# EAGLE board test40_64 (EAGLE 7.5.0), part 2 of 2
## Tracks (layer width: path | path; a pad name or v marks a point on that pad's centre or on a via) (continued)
L2 (continued)
  Top 0.51: J18.2 194.4,280.52 195.75,281.88 324.5,281.88 328,278.38 330,278.38 331.12,279.5 331.49,279.5 J9.2
L3
  Top 0.406: X1.12 26.01,253.89 56.25,284.12 108.12,284.12 114.62,277.62 115.73,277.62 J7.3 116.57,277.57 117.88,278.88 126,278.88 127.12,277.75 127.7,277.75 J17.3 128.44,277.69 129.75,279 178,279 179.25,277.75 180.21,277.75 J8.3 181.05,277.68 182.38,279 189.75,279 191,277.75 191.78,277.75 J18.3
  Top 0.506: J9.3 329.88,277.12 331.12,278.38 340,278.38 341.25,277.12 J19.3 342.88,277.12 344.12,278.38 345.5,278.38 348,280.88 475.38,280.88 478.62,277.62 479.86,277.62 J10.3 480.58,277.7 482,279 490,279 491.38,277.62 492.06,277.62 J20.3
  Top 0.51: J18.3 192.55,277.68 193.88,279 195.12,279 197.12,281 242.88,281 245,278.88 325.88,278.88 327.62,277.12 J9.3
L4
  Top 0.406: X1.31 26.37,252.49 30.12,256.25 30.25,256.25 57,283 107.88,283 114.5,276.38 116.5,276.38 117.75,277.62 118.27,277.62 J7.4 126.06,277.57 127.25,276.38 128.25,276.38 129.5,277.62 130.22,277.62 J17.4 177.93,277.69 179.25,276.38 180.88,276.38 182.12,277.62 182.78,277.62 J8.4 189.7,277.68 191,276.38 192.38,276.38 193.62,277.62 194.35,277.62 J18.4
  Top 0.506: J9.4 340,277.12 341.25,275.88 343.12,275.88 344.25,277 344.73,277 J19.4 346.38,277.12 347.75,278.5 408.25,278.5 408.38,278.38 476.25,278.38 478.25,276.38 480.62,276.38 481.88,277.62 482.39,277.62 J10.4 482.52,277.75 489.88,277.75 491.25,276.38 493.12,276.38 494.45,277.7 J20.4
  Top 0.51: J9.4 331.12,277.12 329.88,275.88 326.25,275.88 325.88,276.25 245.38,276.25 243.88,277.75 194.47,277.75 J18.4
L5
  Top 0.406: X1.13 26.5,251.12 57.5,282.12 107.25,282.12 114.25,275.12 115.69,275.12 J7.5 116.41,275.03 117.62,276.25 126.12,276.25 127.25,275.12 127.72,275.12 J17.5 128.53,275.15 129.88,276.5 178,276.5 179.38,275.12 J8.5 180.88,275.13 182.12,276.38 189.62,276.38 190.88,275.12 J18.5
  Top 0.506: J9.5 329.83,274.58 331.12,275.88 340.12,275.88 341.5,274.5 342.23,274.5 J19.5 342.35,274.62 343.12,274.62 344.38,275.88 477,275.88 477.71,275.17 J10.5 480.67,275.17 481.88,276.38 489.75,276.38 490.88,275.25 492.05,275.25 J20.5
  Top 0.51: J18.5 192.26,275.13 193.5,276.38 242.5,276.38 245.12,273.75 262,273.75 263.12,274.88 325.88,274.88 326.25,274.5 329.02,274.5 J9.5
L6
  Top 0.406: X1.32 26.72,249.72 56.5,279.5 79.25,279.5 79.38,279.38 108.75,279.38 114.5,273.62 116.25,273.62 117.62,275 118.3,275 J7.6 126.09,275.03 127.25,273.88 128.5,273.88 129.62,275 130.14,275 J17.6 178.09,275.15 179.38,273.88 181,273.88 182.25,275.12 182.81,275.12 J8.6 189.49,275.13 190.75,273.88 192.25,273.88 193.38,275 194.26,275 J18.6
  Top 0.506: J9.6 340.17,274.58 341.5,273.25 343,273.25 344.25,274.5 344.76,274.5 J19.6 407.42,274.58 408.75,273.25 427.88,273.25 428.5,273.88 480.75,273.88 482,275.12 482.44,275.12 J10.6 489.58,275.17 490.88,273.88 492.88,273.88 494.12,275.12 494.63,275.12 J20.6
  Top 0.51: J9.6 331.21,274.58 330,273.38 264.38,273.38 262.25,271.25 245.5,271.25 241.62,275.12 J18.6
L7
  Top 0.406: X1.14 27.35,248.35 55.88,277.12 109.62,276.88 114,272.5 115.78,272.5 J7.7 116.36,272.49 117.62,273.75 126,273.75 127.12,272.62 127.75,272.62 J17.7 128.49,272.62 129.75,273.88 178.12,273.88 179.5,272.5 180.19,272.5 J8.7 181.09,272.6 182.38,273.88 189.62,273.88 190.88,272.62 191.83,272.62 J18.7
  Top 0.506: J9.7 329.8,272.05 331,273.25 340.25,273.25 341.5,272 342.26,272 J19.7 343.05,272.05 344.25,273.25 406.38,273.25 408.88,270.75 427,270.75 428.62,272.38 479.69,272.38 J10.7 480.62,272.62 481.88,273.88 489.62,273.88 490.88,272.62 J20.7
  Top 0.51: J18.7 192.34,272.6 193.62,273.88 240,273.88 245.25,268.62 262.38,268.62 265.88,272.12 329.03,272.12 J9.7
L8
  Top 0.406: X1.33 27.23,246.98 54.75,274.5 110,274.5 113.38,271.12 116.5,271.12 117.75,272.38 118.21,272.38 J7.8 126.01,272.49 127.12,271.38 128.38,271.38 129.62,272.62 130.28,272.62 J17.8 178.13,272.62 179.5,271.25 180.75,271.25 182,272.5 182.73,272.5 J8.8 189.53,272.6 190.88,271.25 192.38,271.25 193.62,272.5 194.31,272.5 J18.8
  Top 0.506: J9.8 340.2,272.05 341.5,270.75 342.88,270.75 344.12,272 344.81,272 J19.8 345.06,272.25 404.25,272.25 408.25,268.25 425.88,268.25 429,271.38 480.75,271.38 482,272.62 J10.8 489.5,272.62 490.88,271.38 492.75,271.38 494.12,272.62 J20.8
  Top 0.51: J9.8 331.17,272.05 329.88,270.75 267.25,270.75 262.62,266.12 245.38,266.12 238.88,272.62 194.43,272.62 J18.8
L9
  Top 0.406: X1.15 27.33,245.58 53.5,271.88 111.38,271.88 113.25,270 115.73,270 J7.9 116.58,269.95 117.88,271.25 126,271.25 127.12,270.12 127.7,270.12 J17.9 128.32,270.07 129.62,271.38 178.12,271.38 179.38,270.12 180.22,270.12 J8.9 180.68,270.06 182,271.38 189.75,271.38 191.12,270 191.81,270 J18.9 | 482,271.38 489.38,271.38 489.5,271.25
  Top 0.506: J9.9 329.88,269.5 331.12,270.75 340.12,270.75 341.38,269.5 J19.9 342.88,269.5 344.12,270.75 403.75,270.75 408.88,265.62 425,265.62 429.38,270 479.85,270 J10.9 480.71,270.08 482,271.38 | 489.5,271.25 490.62,270.12 492.1,270.12 J20.9
  Top 0.51: J18.9 192.43,270.06 193.75,271.38 237.25,271.38 245,263.62 261.88,263.62 267.75,269.5 J9.9
L10
  Top 0.406: X1.34 27.34,244.21 52.75,269.5 112,269.25 112.62,268.62 116.38,268.62 117.62,269.88 118.25,269.88 J7.10 126.05,269.95 127.12,268.88 128.25,268.88 129.5,270.12 130.25,270.12 J17.10 178.18,270.07 179.5,268.75 180.75,268.75 182,270 182.77,270 J8.10 189.82,270.06 191.12,268.75 192.25,268.75 193.5,270 194.34,270 J18.10
  Top 0.506: J9.10 340,269.5 341.25,268.25 342.88,268.25 344.12,269.5 J19.10 402.62,269.5 409,263.12 425.25,263.12 430.88,268.75 480.62,268.75 481.96,270.08 J10.10 489.29,270.08 490.5,268.88 493.46,268.88 J20.10
  Top 0.51: J9.10 331.13,269.5 329.88,268.25 268.38,268.25 261.12,261 245.62,261 236.38,270.25 194.59,270.25 J18.10
L11
  Top 0.406: X1.16 27.71,242.84 51.75,266.88 86.25,266.88 86.88,267.5 115.69,267.5 J7.11 116.53,267.41 117.75,268.62 126.12,268.62 127.25,267.5 127.72,267.5 J17.11 128.28,267.54 129.5,268.75 178.25,268.75 179.38,267.62 180.18,267.62 J8.11 181.01,267.51 182.25,268.75 189.88,268.75 191.12,267.5 191.84,267.5 J18.11
  Top 0.506: J9.11 329.84,266.96 331.12,268.25 340,268.25 341.25,267 342.27,267 J19.11 342.84,266.96 344.12,268.25 401.12,268.25 408.88,260.62 425.25,260.62 432.12,267.5 479.89,267.5 J10.11 480.67,267.55 482,268.88 489.25,268.88 490.75,267.38 491.96,267.38 J20.11
  Top 0.51: J18.11 192.39,267.51 193.62,268.75 235,268.75 245.25,258.5 261.12,258.5 269.62,267 329.07,267 J9.11
L12
  Top 0.406: X1.35 28.19,241.44 51,264.25 85.75,264.25 87.62,266.12 116.38,266.12 117.62,267.38 118.29,267.38 J7.12 126.09,267.41 127.25,266.25 128.5,266.25 129.75,267.5 130.26,267.5 J17.12 178.22,267.54 179.5,266.25 180.88,266.25 182.12,267.5 182.81,267.5 J8.12 189.74,267.51 191,266.25 192.38,266.25 193.5,267.38 194.26,267.38 J18.12
  Top 0.506: J9.12 339.91,266.96 341.12,265.75 343,265.75 344.25,267 344.81,267 J19.12 399.91,266.96 408.75,258.12 421.12,258.12 421.25,258 424.75,258 432.88,266.38 479,266.38 479.12,266.25 480.62,266.25 481.75,267.38 482.31,267.38 J10.12 489.2,267.55 490.5,266.25 492.62,266.25 493.75,267.38 494.5,267.38 J20.12
  Top 0.51: J9.12 331.21,266.96 330,265.75 271.12,265.75 261.38,256 244.62,256 233.12,267.5 194.41,267.5 J18.12
L13
  Top 0.406: X1.17 28.45,240.07 50.12,261.75 85.62,261.75 88.5,264.62 115.54,264.62 J7.13 116.37,264.87 117.62,266.12 126.25,266.12 127.25,265.12 127.62,265.12 J17.13 128.5,265 129.75,266.25 178.12,266.25 179.25,265.12 180.13,265.12 J8.13 180.72,264.98 182,266.25 189.88,266.25 191.12,265 191.84,265 J18.13
  Top 0.506: J9.13 329.93,264.43 331.25,265.75 339.75,265.75 341.12,264.38 342.26,264.38 J19.13 342.38,264.5 342.88,264.5 344,265.62 398.75,265.62 408.88,255.5 425,255.5 434.5,265 J10.13 480.63,265 481.88,266.25 489.12,266.25 490.38,265 J20.13
  Top 0.51: J18.13 192.47,264.98 193.75,266.25 232.12,266.25 245,253.38 261.62,253.38 272.5,264.25 328.94,264.25 J9.13
L14
  Top 0.406: X1.36 28.45,238.7 49,259.25 85.5,259.25 89.88,263.62 116.38,263.62 117.5,264.75 118.2,264.75 J7.14 126,264.87 127.12,263.75 128.62,263.75 129.75,264.88 130.18,264.88 J17.14 178,265 179.25,263.75 181,263.75 182.12,264.88 182.72,264.88 J8.14 189.78,264.98 191,263.75 192.5,263.75 193.62,264.88 193.88,264.88 194.3,264.88 J18.14
  Top 0.506: J9.14 339.95,264.43 341.25,263.12 342.88,263.12 344.12,264.38 344.8,264.38 J19.14 397.32,264.43 408.75,253 425.38,253 436.12,263.75 480.62,263.75 481.88,265 J10.14 489,265 490.25,263.75 492.75,263.75 494,265 J20.14
  Top 0.51: J9.14 331.18,264.43 329.88,263.12 274,263.12 261.75,250.88 245.5,250.88 231.5,264.88 193.88,264.88
L15
  Top 0.406: X1.18 28.8,237.3 48.25,256.75 84.75,256.75 90.25,262.25 115.7,262.25 J7.15 116.45,262.33 117.75,263.62 126,263.62 127.12,262.5 127.71,262.5 J17.15 128.58,262.45 129.88,263.75 177.88,263.75 179.12,262.5 180.22,262.5 J8.15 180.94,262.44 182.25,263.75 189.75,263.75 191,262.5 191.79,262.5 J18.15
  Top 0.506: J9.15 329.76,261.88 331,263.12 340,263.12 341.25,261.88 J19.15 342.88,261.88 344.25,263.25 396,263.25 408.75,250.5 425.25,250.5 437.21,262.46 J10.15 480.59,262.46 481.88,263.75 489,263.75 490.12,262.62 491.98,262.62 J20.15
  Top 0.51: J18.15 192.44,262.44 193.75,263.75 229.88,263.75 245.25,248.38 261.38,248.38 275,262 329,262 J9.15
L16
  Top 0.406: X1.37 29.05,235.93 47.25,254.12 84.5,254.12 91.5,261.12 116.62,261.12 117.88,262.38 118.28,262.38 J7.16 125.92,262.33 127.12,261.12 128.25,261.12 129.5,262.38 130.22,262.38 J17.16 178.17,262.45 179.5,261.12 180.75,261.12 182,262.38 182.76,262.38 J8.16 189.81,262.44 191.12,261.12 192.62,261.12 193.75,262.25 194.22,262.25 J18.16
  Top 0.506: J9.16 339.99,261.88 341.25,260.62 342.88,260.62 344.12,261.88 J19.16 394.87,261.88 408.88,247.88 425,247.88 438.25,261.12 480.5,261.12 481.75,262.38 482.38,262.38 J10.16 489.04,262.46 490.25,261.25 492.88,261.25 494.12,262.5 494.64,262.5 J20.16
  Top 0.51: J9.16 331.13,261.88 329.88,260.62 276.38,260.62 261.62,245.88 245,245.88 228.5,262.38 194.46,262.38 J18.16
L17
  Top 0.406: X2.11 24.01,185.51 28.12,189.62 28.12,232.25 47.5,251.62 84.62,251.62 92.5,259.5 115.5,259.5 J7.17 116.54,259.79 117.75,261 126.12,261 127.12,260 127.67,260 J17.17 128.29,259.92 129.5,261.12 178.25,261.12 179.5,259.88 180.26,259.88 J8.17 180.9,259.89 182.12,261.12 189.88,261.12 191.12,259.88 191.84,259.88 J18.17
  Top 0.506: J9.17 329.85,259.35 331.12,260.62 340,260.62 341.38,259.25 342.21,259.25 J19.17 342.34,259.38 342.88,259.38 344.12,260.62 393.88,260.62 409.12,245.38 425.12,245.38 439.68,259.93 J10.17 480.55,259.93 481.88,261.25 489,261.25 490.38,259.88 492.08,259.88 J20.17
  Top 0.51: J18.17 192.52,259.89 193.75,261.12 227.25,261.12 245.12,243.25 261.5,243.25 277.5,259.25 329.01,259.25 J9.17
L18
  Top 0.406: X2.30 24.27,184.14 29.12,189 29.12,231.38 46.75,249 84.38,249 93.88,258.5 116.38,258.5 117.75,259.88 118.24,259.88 J7.18 125.96,259.79 127.12,258.62 128.38,258.62 129.62,259.88 130.25,259.88 J17.18 178.09,259.92 179.38,258.62 181,258.62 182.25,259.88 182.81,259.88 J8.18 189.73,259.89 191,258.62 192.38,258.62 193.62,259.88 194.38,259.88 J18.18
  Top 0.506: J9.18 339.9,259.35 341.12,258.12 343,258.12 344.12,259.25 344.75,259.25 J19.18 344.94,259.25 392.25,259.25 408.62,242.88 425,242.88 440.75,258.62 480.5,258.62 481.8,259.93 J10.18 488.95,259.93 490.25,258.62 492.62,258.62 493.88,259.88 494.62,259.88 J20.18
  Top 0.51: J9.18 331.22,259.35 330,258.12 278.75,258.12 261.38,240.75 245.25,240.75 226.25,259.75 194.54,259.75 J18.18
L19
  Top 0.406: X2.12 24.39,182.77 30,188.38 30,230.75 45.75,246.5 84.25,246.5 95,257.25 J7.19 116.38,257.25 117.62,258.5 126,258.5 127.12,257.38 J17.19 128.5,257.38 129.75,258.62 178,258.62 179.25,257.38 180.26,257.38 J8.19 180.85,257.36 182.12,258.62 189.88,258.62 191.12,257.38 191.84,257.38 J18.19
  Top 0.506: J9.19 329.93,256.81 331.25,258.12 339.75,258.12 341.12,256.75 342.25,256.75 J19.19 342.93,256.81 344.25,258.12 390.62,258.12 408.5,240.25 425.38,240.25 442.62,257.5 479.82,257.5 J10.19 | 479.93,257.38 J10.19 | J10.19 480.51,257.38 481.75,258.62 489,258.62 490.25,257.38 J20.19
  Top 0.51: J18.19 192.23,257.36 193.5,258.62 224.62,258.62 245.12,238.12 261.62,238.12 280.38,256.88 329.04,256.88 J9.19
L20
  Top 0.406: X2.31 24.5,181.37 31.25,188.12 31.25,230.38 44.75,243.88 44.88,243.88 45,244 85.38,244 96.75,255.38 96.88,255.38 97.5,256 116.5,256 117.75,257.25 J7.20 126,257.25 127.12,256.12 128.5,256.12 129.62,257.25 130.17,257.25 J17.20 177.88,257.38 179.25,256 180.62,256 182,257.38 182.81,257.38 J8.20 189.9,257.36 191.25,256 192.25,256 193.5,257.25 194.29,257.25 J18.20
  Top 0.506: J9.20 339.94,256.81 341.25,255.5 343,255.5 344.25,256.75 344.8,256.75 J19.20 344.9,256.75 389.38,256.75 408.38,237.75 425.25,237.75 443.62,256.12 480.62,256.12 481.88,257.38 J10.20 488.87,257.38 490.12,256.12 492.75,256.12 493.88,257.25 494.54,257.25 J20.20
  Top 0.51: J9.20 331.18,256.81 329.88,255.5 281.12,255.5 261.25,235.62 245.25,235.62 223.62,257.25 194.5,257.25 J18.20
L21
  Top 0.406: X2.13 24.5,180 32,187.5 32,229.38 43.88,241.38 44,241.38 44.12,241.5 79.88,241.5 80,241.38 84.5,241.38 97.88,254.75 115.75,254.75 J7.21 116.33,254.71 117.62,256 126.12,256 127.12,255 127.59,255 J17.21 128.46,254.84 129.62,256 178,256 179.12,254.88 180.22,254.88 J8.21 180.81,254.81 182,256 189.75,256 191,254.75 191.79,254.75 J18.21
  Top 0.506: J9.21 329.89,254.26 331.12,255.5 340,255.5 341.25,254.25 342.3,254.25 J19.21 343.01,254.26 344.25,255.5 388,255.5 408.25,235.25 425.25,235.25 444.75,254.75 479.84,254.75 J10.21 480.6,254.84 481.88,256.12 488.75,256.12 490,254.88 492.11,254.88 J20.21
  Top 0.51: J18.21 192.19,254.81 193.38,256 222.25,256 245.12,233.12 261.5,233.12 282.75,254.38 329,254.38 J9.21
L22
  Top 0.406: X2.32 24.85,178.6 33.25,187 33.25,229 43.25,239 66.88,239 67,238.88 84.25,238.88 98.88,253.5 116.5,253.5 117.71,254.71 J7.22 126.04,254.71 127.25,253.5 128.5,253.5 129.75,254.75 130.21,254.75 J17.22 177.29,254.84 178.62,253.5 180.88,253.5 182,254.62 182.63,254.62 J8.22 189.69,254.81 191,253.5 192.25,253.5 193.5,254.75 194.34,254.75 J18.22
  Top 0.506: J9.22 339.86,254.26 341.12,253 343.12,253 344.25,254.12 344.71,254.12 J19.22 344.99,254.12 387.12,254.12 408.62,232.62 425.25,232.62 446.25,253.62 480.62,253.62 481.85,254.84 J10.22 488.53,254.84 489.75,253.62 492.75,253.62 494,254.88 494.64,254.88 J20.22
  Top 0.51: J9.22 331.01,254.26 329.75,253 283.62,253 261.25,230.62 261.12,230.62 261,230.5 245.62,230.5 221.25,254.88 194.46,254.88 J18.22
L23
  Top 0.406: X2.14 24.98,177.23 34.62,186.88 34.62,228.5 42.5,236.38 79.12,236.38 79.25,236.25 84.12,236.25 100,252.12 115.74,252.12 J7.23 116.3,252.17 117.5,253.38 126.25,253.38 127.33,252.29 J17.23 128.42,252.29 129.62,253.5 177.5,253.5 178.75,252.25 180.26,252.25 J8.23 180.9,252.28 182.12,253.5 189.88,253.5 191.12,252.25 191.84,252.25 J18.23 | J19.23 343.1,251.72 344.38,253 345.88,253
  Top 0.506: J9.23 329.73,251.72 331,253 339.75,253 341,251.75 342.29,251.75 J19.23 | 345.88,253 385.88,253 408.75,230.12 425.5,230.12 447.62,252.25 479.88,252.25 J10.23 480.56,252.31 481.75,253.5 488.5,253.5 489.75,252.25 492.08,252.25 J20.23
  Top 0.51: J18.23 192.4,252.28 193.62,253.5 219.75,253.5 245.25,228 261,228 284.62,251.75 328.96,251.88 J9.23
L24
  Top 0.406: X2.33 24.98,175.86 35.62,186.5 35.62,228 41.38,233.75 84.88,233.75 102,250.88 116.38,250.88 117.75,252.25 118.25,252.25 J7.24 126.08,252.17 127.38,250.88 128.12,250.88 129.38,252.12 130.12,252.12 J17.24 176.83,252.29 178.12,251 180.88,251 182.12,252.25 182.8,252.25 J8.24 189.72,252.28 191,251 192.62,251 193.75,252.12 194.25,252.12 J18.24
  Top 0.506: J9.24 339.65,251.72 341,250.38 342.75,250.38 344,251.62 344.75,251.62 J19.24 384.52,251.72 408.62,227.62 426,227.62 449.5,251.12 478.88,251.12 479,251 480.62,251 481.88,252.25 482.42,252.25 J10.24 488.44,252.31 489.75,251 492.75,251 494,252.25 494.62,252.25 J20.24
  Top 0.51: J9.24 330.98,251.72 329.75,250.5 286.12,250.5 261.12,225.5 245,225.5 218.38,252.12 194.55,252.12 J18.24
L25
  Top 0.406: X2.15 25.21,174.46 37.5,186.75 37.5,228.12 40.5,231.12 84.75,231.12 103.25,249.62 J7.25 116.38,249.63 117.62,250.88 125.88,250.88 127,249.75 J17.25 128.25,249.75 129.5,251 176.88,251 178.25,249.62 180.18,249.62 J8.25 180.86,249.74 182.12,251 189.62,251 190.88,249.75 191.84,249.75 J18.25
  Top 0.506: J9.25 329.69,249.19 330.88,250.38 339.62,250.38 340.88,249.12 342.25,249.12 J19.25 342.81,249.19 344,250.38 383.38,250.38 408.75,225 425.62,225 450,249.38 479.55,249.38 J10.25 480.64,249.76 481.88,251 488.38,251 489.62,249.75 J20.25
  Top 0.51: J18.25 192.49,249.74 193.75,251 217,251 245.12,222.88 261.5,222.88 287.62,249 328.93,249 J9.25
L26
  Top 0.406: X2.34 25.59,173.09 38.62,186.12 38.62,227 41.38,229.75 41.5,229.75 41.88,230.12 85.5,230.12 103.75,248.38 116.5,248.38 117.75,249.62 J7.26 125.87,249.63 127,248.5 128.25,248.5 129.38,249.62 130.16,249.62 J17.26 176.87,249.75 178.12,248.5 181,248.5 182.25,249.75 182.81,249.75 J8.26 189.51,249.74 190.75,248.5 192.38,248.5 193.5,249.62 194.29,249.62 J18.26
  Top 0.506: J9.26 339.44,249.19 340.75,247.88 343,247.88 344.25,249.12 344.79,249.12 J19.26 344.91,249.12 382.25,249.12 408.88,222.5 425.5,222.5 451.5,248.5 480.75,248.5 482.01,249.76 J10.26 488.24,249.76 489.5,248.5 492.62,248.5 493.88,249.75 J20.26
  Top 0.51: J9.26 331.06,249.19 329.75,247.88 288.62,247.88 261.12,220.38 244.75,220.38 215.5,249.62 194.51,249.62 J18.26
L27
  Top 0.406: X2.16 35.97,171.72 111.38,247.12 115.75,247.12 J7.27 116.59,247.09 117.75,248.25 126.12,248.25 127.12,247.25 127.72,247.25 J17.27 128.22,247.22 129.5,248.5 177,248.5 178.25,247.25 180.23,247.25 J8.27 180.94,247.19 182.25,248.5 189.62,248.5 190.88,247.25 191.81,247.25 J18.27
  Top 0.506: J9.27 329.77,246.65 331,247.88 339.5,247.88 340.75,246.62 342.29,246.62 J19.27 343.02,246.65 344.25,247.88 380.88,247.88 408.75,220 425.5,220 452.88,247.38 479.79,247.38 J10.27 480.73,247.22 482,248.5 488.12,248.5 489.5,247.12 492.04,247.12 J20.27
  Top 0.51: J18.27 192.32,247.19 193.62,248.5 213.75,248.5 244.88,217.38 261,217.38 290.25,246.62 329.09,246.62 J9.27
L28
  Top 0.406: X2.35 35.82,170.32 111.38,245.88 116.62,245.88 117.75,247 118.23,247 J7.28 126.03,247.09 127.12,246 128.25,246 129.5,247.25 130.26,247.25 J17.28 177.16,247.22 178.5,245.88 180.88,245.88 182.25,247.25 182.77,247.25 J8.28 189.56,247.19 190.88,245.88 192.38,245.88 193.62,247.12 194.33,247.12 J18.28
  Top 0.506: J9.28 339.48,246.65 340.75,245.38 343,245.38 344.25,246.62 344.83,246.62 J19.28 344.87,246.62 379.5,246.62 408.75,217.38 425.12,217.38 425.25,217.5 425.38,217.5 453.75,245.88 480.5,245.88 480.62,246 480.75,246 481.98,247.22 J10.28 488.15,247.22 489.38,246 492.75,246 494,247.25 494.65,247.25 J20.28
  Top 0.51: J9.28 331.02,246.65 329.75,245.38 291,245.38 261.62,216 244,216 212.88,247.12 194.47,247.12 J18.28
L29
  Top 0.406: X2.17 35.95,168.95 111.62,244.62 115.71,244.62 J7.29 116.55,244.55 117.75,245.75 126.25,245.75 127.25,244.75 127.68,244.75 J17.29 128.3,244.68 129.5,245.88 177.38,245.88 178.62,244.62 180.25,244.62 J8.29 180.78,244.66 182,245.88 189.5,245.88 190.75,244.62 191.83,244.62 J18.29
  Top 0.506: J9.29 329.73,244.1 331,245.38 339.5,245.38 340.75,244.12 342.29,244.12 J19.29 343.11,244.1 344.38,245.38 378,245.38 408.5,214.88 425.12,214.88 453.62,243.38 453.62,243.5 454.62,244.5 479.75,244.5 J10.29 480.69,244.69 482,246 488.12,246 489.38,244.75 492.07,244.75 J20.29
  Top 0.51: J18.29 192.41,244.66 193.62,245.88 212.38,245.88 243.38,214.88 262.38,214.88 291.62,244.12 329.09,244.12 J9.29
L30
  Top 0.406: X2.36 35.95,167.58 111.5,243.25 116.25,243.25 117.5,244.5 118.28,244.5 J7.30 125.95,244.55 127.12,243.38 128.25,243.38 129.5,244.62 130.25,244.62 J17.30 177.2,244.68 178.5,243.38 180.88,243.38 182.12,244.62 182.79,244.62 J8.30 189.47,244.66 190.75,243.38 192.5,243.38 193.62,244.5 194.25,244.5 J18.30
  Top 0.506: J9.30 339.39,244.1 340.62,242.88 343.12,242.88 344.25,244 344.75,244 J19.30 344.95,244 377,244 382.25,238.75 382.38,238.75 408.75,212.38 425.12,212.38 456.12,243.38 480.62,243.38 481.94,244.69 J10.30 487.94,244.69 489.25,243.38 492.75,243.38 494,244.62 494.62,244.62 J20.30
  Top 0.51: J9.30 331.11,244.1 329.88,242.88 292.25,242.88 262.88,213.5 243,213.5 211.75,244.75 194.5,244.75 J18.30
L31
  Top 0.406: X2.18 35.81,166.18 111.62,242 115.78,242 J7.31 116.26,242.01 117.5,243.25 126,243.25 127.12,242.12 127.75,242.12 J17.31 128.38,242.13 129.62,243.38 177.12,243.38 178.38,242.12 J8.31 180.74,242.12 182,243.38 189.38,243.38 190.62,242.12 J18.31
  Top 0.506: J9.31 329.81,241.56 331.12,242.88 339.38,242.88 340.62,241.62 342.25,241.62 J19.31 343.06,241.56 344.38,242.88 375.5,242.88 408.5,209.88 425.5,209.88 457.75,242.12 479.92,242.12 J10.31 480.52,242.15 481.75,243.38 488,243.38 489.25,242.12 492.12,242.12 J20.31
  Top 0.51: J18.31 192.49,242.12 193.75,243.38 206.88,243.38 243.62,206.62 261.88,206.62 295.75,240.5 295.88,240.5 296.88,241.5 329.05,241.5 J9.31
L32
  Top 0.406: X2.37 35.94,164.81 112.12,240.75 116.38,240.75 117.62,242 118.31,242 J7.32 125.86,242.01 127,240.88 128.25,240.88 129.38,242 130.16,242 J17.32 176.87,242.13 178.25,240.75 180.62,240.75 181.88,242 182.71,242 J8.32 189.38,242.12 190.75,240.75 192.38,240.75 193.5,241.88 194.16,241.88 J18.32
  Top 0.506: J9.32 339.19,241.56 340.5,240.25 342.88,240.25 344.12,241.5 344.79,241.5 J19.32 374.31,241.56 408.62,207.25 425.62,207.25 459.25,240.88 480.5,240.88 481.75,242.12 482.45,242.12 J10.32 488.11,242.15 489.38,240.88 492.88,240.88 494.12,242.12 494.65,242.12 J20.32
  Top 0.51: J9.32 331.19,241.56 330,240.38 329.88,240.38 329.75,240.25 297.25,240.25 262.5,205.5 243.12,205.5 206.62,242 194.51,242 J18.32
L33
  Top 0.406: X3.11 20.88,115.06 20.88,115.62 22.5,117.25 23.88,117.25 31.75,125.12 31.75,159.5 112.22,239.47 J7.33 116.47,239.47 117.75,240.75 126.12,240.75 127.25,239.62 127.72,239.62 J17.33 128.34,239.59 129.5,240.75 177.12,240.75 178.25,239.62 180.24,239.62 J8.33 180.7,239.57 181.88,240.75 189.25,240.75 190.38,239.62 191.81,239.62 J18.33
  Top 0.506: J9.33 329.9,239.03 331.12,240.25 339.12,240.25 340.38,239 342.29,239 J19.33 342.54,239.25 343.12,239.25 344.12,240.25 372.62,240.25 408.5,204.38 424.88,204.38 460.11,239.6 J10.33 480.36,239.6 481.62,240.88 488.12,240.88 489.38,239.62 492.12,239.62 J20.33
  Top 0.51: J18.33 192.32,239.57 193.5,240.75 206.12,240.75 242.38,204.5 263.12,204.5 269.5,210.88 269.62,210.88 297.62,238.88 328.96,238.88 J9.33
L34
  Top 0.406: X3.30 32.75,122.72 32.75,159.12 111.88,238.25 116.62,238.25 117.84,239.47 J7.34 126.03,239.47 127.12,238.38 128.38,238.38 129.5,239.5 130.2,239.5 J17.34 177.03,239.59 178.25,238.38 181,238.38 182.12,239.5 182.75,239.5 J8.34 189.05,239.57 190.25,238.38 192.75,238.38 193.75,239.38
  Top 0.506: J9.34 338.73,239.03 340,237.75 342.88,237.75 344.12,239 344.82,239 J19.34 372.23,239.03 408,203.25 425.88,203.25 461,238.38 480.62,238.38 481.75,239.5 482.37,239.5 J10.34 488.02,239.6 489.25,238.38 492.75,238.38 493.88,239.5 494.57,239.5 J20.34
  Top 0.51: J9.34 331.15,239.03 329.88,237.75 298.25,237.75 297.75,237.25 297.62,237.25 263.88,203.5 241.5,203.5 205.5,239.5 194.47,239.5 J18.34 194.2,239.38 193.75,239.38
L35
  Top 0.406: X3.12 20.23,111.62 24.5,111.62 33.75,120.88 33.75,158.88 111.81,236.93 J7.35 116.56,236.93 117.75,238.12 126.12,238.12 127.12,237.12 127.69,237.12 J17.35 128.43,237.06 129.75,238.38 176.88,238.38 178.25,237 180.25,237 J8.35 181.03,237.03 182.25,238.25 189.25,238.25 190.5,237 191.82,237 J18.35
  Top 0.506: J9.35 329.74,236.49 331,237.75 338.75,237.75 340,236.5 342.3,236.5 J19.35 342.32,236.5 343,236.5 344.25,237.75 371.38,237.75 407,202.12 426.88,202.12 461.81,237.06 J10.35 480.56,237.06 481.88,238.38 488,238.38 489.25,237.12 492.07,237.12 J20.35
  Top 0.51: J18.35 192.53,237.03 193.88,238.38 205,238.38 241,202.38 264.62,202.38 298.62,236.38 329,236.38 J9.35
L36
  Top 0.406: X3.31 24.62,110.25 34.75,120.38 34.75,158.75 111.62,235.62 116.38,235.62 117.68,236.93 J7.36 125.94,236.93 127,235.88 128.62,235.88 129.75,237 130.24,237 J17.36 176.69,237.06 178,235.75 181,235.75 182.25,237 182.79,237 J8.36 189.09,237.03 190.38,235.75 192.25,235.75 193.5,237 194.37,237 J18.36
  Top 0.506: J9.36 338.26,236.49 339.5,235.25 343,235.25 344.12,236.38 344.74,236.38 J19.36 371.01,236.49 406.5,201 427.62,201 462.38,235.75 480.5,235.75 481.88,237.12 482.42,237.12 J10.36 487.94,237.06 489.25,235.75 492.88,235.75 494.12,237 494.61,237 J20.36
  Top 0.51: J9.36 330.99,236.49 329.75,235.25 299.12,235.25 265.25,201.38 240.12,201.38 204.5,237 194.44,237 J18.36
L37
  Top 0.406: X3.13 24.75,108.88 35.75,119.88 35.75,158.5 111.64,234.39 J7.37 116.14,234.39 117.38,235.62 126,235.62 127.12,234.5 127.74,234.5 J17.37 128.64,234.51 129.88,235.75 176.5,235.62 177.62,234.5 J8.37 181,234.5 182.12,235.62 188.88,235.62 190,234.5 J18.37
  Top 0.506: J9.37 329.82,233.94 331.12,235.25 338.12,235.25 339.38,234 342.25,234 J19.37 342.49,234.12 343,234.12 344.12,235.25 370.5,235.25 405.75,200 428.25,200 462.77,234.53 J10.37 480.52,234.53 481.75,235.75 488,235.75 489.25,234.5 492.11,234.5 J20.37
  Top 0.51: J18.37 192.25,234.5 193.5,235.75 204,235.75 239.5,200.25 265.88,200.25 292.12,226.5 292.12,226.62 299.38,233.88 329.04,233.88 J9.37
L38
  Top 0.406: X3.32 23.07,107.5 24.75,107.5 36.75,119.5 36.75,158.12 111.75,233.12 116.5,233.12 117.77,234.39 J7.38 125.48,234.39 126.75,233.12 128.5,233.12 129.75,234.38 130.16,234.38 J17.38 175.99,234.51 177.25,233.25 180.88,233.25 182,234.38 182.71,234.38 J8.38 188.88,234.5 190.12,233.25 192.25,233.25 193.5,234.5 J18.38
  Top 0.506: J9.38 338.31,233.94 339.62,232.62 342.88,232.62 344.12,233.88 344.78,233.88 J19.38 370.18,233.94 405.25,198.88 429.12,198.88 463.5,233.25 480.62,233.25 481.88,234.5 482.45,234.5 J10.38 487.73,234.53 489,233.25 492.88,233.25 494.12,234.5 J20.38
  Top 0.51: J9.38 331.19,233.94 330,232.75 300,232.75 266.25,199 238.75,199 203.25,234.5 J18.38
L39
  Top 0.406: X3.14 20.22,106.12 24.88,106.12 37.88,119.12 37.88,157.75 111.97,231.85 J7.39 116.47,231.85 117.75,233.12 125.62,233.12 126.75,232 127.73,232 J17.39 128.47,231.97 129.75,233.25 176.25,233.25 177.5,232 180.24,232 J8.39 180.58,231.96 181.88,233.25 189,233.25 190.25,232 191.81,232 J18.39
  Top 0.506: J9.39 329.9,231.41 331.12,232.62 338.25,232.62 339.5,231.38 342.28,231.38 J19.39 342.4,231.5 343,231.5 344.12,232.62 369.5,232.62 404.38,197.75 429.75,197.75 463.99,231.99 J10.39 480.61,231.99 481.88,233.25 487.62,233.25 489,231.88 492.02,231.88 J20.39
  Top 0.51: J18.39 192.33,231.96 193.5,233.12 203,233.12 238.25,197.88 267,197.88 292.88,223.75 293,223.75 300.62,231.38 329.08,231.38 J9.39
L40
  Top 0.406: X3.33 23.19,104.88 25,104.88 39,118.88 39,157.5 112.12,230.62 116.5,230.62 117.72,231.85 J7.40 119.53,231.85 121,230.38 128.5,230.38 129.5,231.38 129.69,231.38 J17.40 175.78,231.97 177,230.75 180.75,230.75 182,232 182.78,232 J8.40 189.04,231.96 190.25,230.75 192.62,230.75 193.75,231.88 194.32,231.88 J18.40
  Top 0.506: J9.40 337.97,231.41 339.25,230.12 343,230.12 344.12,231.25 344.69,231.25 J19.40 368.85,231.41 403.75,196.5 430.38,196.5 464.5,230.75 480.75,230.75 481.88,231.88 482.37,231.88 J10.40 487.39,231.99 488.62,230.75 493,230.75 494.12,231.88 494.56,231.88 J20.40
  Top 0.51: J9.40 331.03,231.41 329.75,230.12 301,230.12 267.75,196.88 237.5,196.88 202.25,232.12 194.57,232.12 J18.40 194.44,232
L41
  Top 0.406: X3.15 24.97,103.34 40.12,118.5 40.12,156.75 112.75,229.38 180.25,229.38 J8.41 180.66,229.41 181.88,230.62 189.12,230.62 190.38,229.38 191.82,229.38 J18.41
  Top 0.506: J9.41 329.87,228.87 331.12,230.12 338,230.12 339.25,228.88 J19.41 343,228.88 344.25,230.12 346,230.12 346.12,230.25 368.25,230.25 403,195.5 431,195.5 464.94,229.44 J10.41 480.69,229.44 482,230.75 487.38,230.75 488.62,229.5 492.08,229.5 J20.41
  Top 0.51: J18.41 192.54,229.41 193.75,230.62 202.5,230.62 237.25,195.88 268.38,195.88 300.5,228 300.62,228 301.5,228.88 J9.41
L42
  Top 0.406: X3.34 24.97,101.97 41.12,118.12 41.12,156.5 113.12,228.5 179,228.5 179.38,228.12 180.75,228.12 182,229.38 182.78,229.38 J8.42 188.96,229.41 190.25,228.12 192.38,228.12 193.5,229.25 194.24,229.25 J18.42 | 339.38,227.5 342.88,227.5 344.25,228.88 J19.42
  Top 0.506: J9.42 338.01,228.87 339.38,227.5 | 344.74,228.75 J19.42 368.13,228.87 402.62,194.38 431.75,194.38 465.5,228.12 480.62,228.12 481.88,229.38 482.4,229.38 J10.42 482.53,229.5 487.12,229.5 488.5,228.12 493.25,228.12 494.57,229.44 J20.42
  Top 0.51: J9.42 331.37,228.87 330.12,227.62 301.75,227.62 269.12,195 236.5,195 202,229.5 194.49,229.5 J18.42 194.44,229.38
L43
  Top 0.406: X3.16 24.97,100.6 42.12,117.75 42.12,156.25 113.38,227.5 178.62,227.5 179.25,226.88 J8.43 180.62,226.88 181.88,228.12 189,228.12 190.25,226.88 J18.43
  Top 0.506: J9.43 329.95,226.32 331.25,227.62 337.88,227.62 339.12,226.38 342.26,226.38 J19.43 342.36,226.38 343,226.38 344.25,227.62 367.75,227.62 402,193.38 432.38,193.38 465.9,226.91 J10.43 480.53,226.91 481.75,228.12 487.25,228.12 488.5,226.88 492.11,226.88 J20.43
  Top 0.51: J18.43 192.5,226.88 193.62,228 193.75,228 193.88,228.12 201.75,228.12 235.88,194 269.75,194 302.12,226.38 329.06,226.38 J9.43
L44
  Top 0.406: X3.35 23.23,99.38 25.12,99.38 43.25,117.5 43.25,156 113.88,226.62 177.12,226.62 178.12,225.62 180.88,225.62 182.12,226.88 J8.44 189.12,226.88 190.38,225.62 192.5,225.62 193.75,226.88 J18.44
  Top 0.506: 329.75,225.12 330.2,225.12 331.4,226.32 J9.44 337.93,226.32 339.25,225 343.12,225 344.38,226.25 344.77,226.25 J19.44 367.55,226.32 401.62,192.25 432.88,192.25 466.25,225.62 480.75,225.62 482,226.88 482.44,226.88 J10.44 487.1,226.91 488.38,225.62 492.88,225.62 494,226.75 494.52,226.75 J20.44
  Top 0.51: 329.75,225.12 302.75,225.12 302.12,224.5 302,224.5 270.38,192.88 235.38,192.88 201.38,226.88 J18.44 194.53,226.75
L45
  Top 0.406: X3.17 25.08,97.83 44.38,117.12 44.38,155.62 114.62,225.88 176.75,225.75 178.12,224.38 180.25,224.38 J8.45 180.71,224.34 182,225.62 189.12,225.62 190.38,224.38 191.82,224.38 J18.45 | J19.45 343.16,223.78 344.38,225
  Top 0.506: J9.45 329.91,223.78 331.12,225 337.62,225 338.88,223.75 342.27,223.75 J19.45 | 344.38,225 367.25,225 401,191.25 433.38,191.25 466.49,224.37 J10.45 480.62,224.37 481.88,225.62 487,225.62 488.25,224.38 J20.45
  Top 0.51: J18.45 192.59,224.34 193.88,225.62 201.12,225.62 234.88,191.88 271,191.88 303.25,224.12 328.77,224.12 J9.45
L46
  Top 0.406: X3.36 25.08,96.46 45.5,116.88 45.5,155.12 110.12,219.75 131.25,219.75 136.38,224.88 176.12,224.88 177.88,223.12 181,223.12 182.12,224.25 182.74,224.25 J8.46 188.91,224.34 190.12,223.12 192.62,223.12 193.75,224.25 193.88,224.25 194.31,224.25 J18.46
  Top 0.506: J9.46 337.59,223.78 338.88,222.5 343.12,222.5 344.38,223.75 344.81,223.75 J19.46 366.84,223.78 400.62,190 433.75,190 466.88,223.12 480.75,223.12 482,224.38 J10.46 486.88,224.37 488.12,223.12 493,223.12 494.12,224.25 494.56,224.25 J20.46
  Top 0.51: J9.46 331.29,223.78 330,222.5 303.25,222.5 271.62,190.88 234.38,190.88 201,224.25 194.49,224.25 J18.46 | 194,224.38 193.88,224.25
L47
  Top 0.406: X3.18 25.31,95.06 46.62,116.38 46.62,154.5 110.38,218.25 131.38,218.25 136.88,223.75 175.75,223.75 177.5,222 180.08,222 J8.47 181.04,221.79 182.38,223.12 188.75,223.12 190.12,221.75 191.81,221.75 J18.47 | J9.47 330,221.25 331.25,222.5 337.75,222.5 339,221.25 J19.47
  Top 0.506: J19.47 342.44,221.38 343.12,221.38 344.25,222.5 366.25,222.5 399.88,188.88 434.25,188.88 467.2,221.82 J10.47 480.7,221.82 482,223.12 486.88,223.12 488.25,221.75 492.06,221.75 J20.47
  Top 0.51: J18.47 192.54,221.79 193.88,223.12 200.62,223.12 233.88,189.88 272.5,189.88 303.88,221.25 J9.47
L48
  Top 0.406: X3.37 23.11,93.75 25.5,93.75 47.62,115.88 47.62,153.75 111,217.12 131.75,217.12 137.38,222.75 175.38,222.75 177.62,220.5 181.25,220.5 182.54,221.79 J8.48 188.83,221.79 190,220.62 192.88,220.62 193.88,221.62 194.23,221.62 J18.48 | J9.48 337.88,221.25 339.12,220 342.88,220 344.12,221.25 J19.48
  Top 0.506: J19.48 366.13,221.25 399.62,187.75 434.5,187.75 467.25,220.5 480.5,220.5 481.75,221.75 482.4,221.75 J10.48 486.93,221.82 488.12,220.62 493,220.62 494.12,221.75 494.6,221.75 J20.48
  Top 0.51: J9.48 331,221.25 329.75,220 304.38,220 273,188.62 233.5,188.62 200.38,221.75 194.44,221.75 J18.48 194.48,221.88
L49
  Top 0.406: 48.88,110.75 48.88,153.12 111.5,215.75 132.25,215.75 135.75,219.25 J8.49 181.13,219.25 182.5,220.62 188.62,220.62 190,219.25 J18.49 | J9.49 329.7,218.71 330.88,219.88 338.12,219.88 339.25,218.75 342.26,218.75 J19.49
  Top 0.506: J19.49 342.83,218.71 344.12,220 365.75,220 399,186.75 435,186.75 467.62,219.38 479.85,219.38 J10.49 480.54,219.28 481.88,220.62 486.75,220.62 488.12,219.25 492.1,219.25 J20.49
  Top 0.51: J18.49 192.63,219.25 193.88,220.5 199.75,220.5 199.88,220.38 200,220.38 232.88,187.5 273.62,187.5 304.88,218.75 329.06,218.75 J9.49 | 48.88,110.75 48.88,73.12 24.5,48.75 20.27,48.75 X4.9
L50
  Top 0.406: 50.12,108.38 50,108.5 50,152.5 112,214.5 132.75,214.5 136,217.75 181.12,217.75 182.63,219.25 J8.50 188.5,219.25 190,217.75 192.12,217.75 | J18.50 | J9.50 338.17,218.71 339.5,217.38 343,217.38 344.25,218.62 344.77,218.62 J19.50
  Top 0.506: J19.50 344.89,218.75 365.62,218.75 398.62,185.75 435.38,185.75 467.62,218 480.62,218 481.91,219.28 J10.50 486.84,219.28 488.12,218 492.62,218 493.75,219.12 494.51,219.12 J20.50
  Top 0.51: 192.12,217.75 192.9,217.75 J18.50 | J9.50 330.95,218.71 329.75,217.5 305.38,217.5 274.25,186.38 232.5,186.38 199.75,219.12 194.53,219.12 J18.50 | J18.50 | 50.12,108.38 50.12,73 24.5,47.38 24,47.38 23.88,47.5 23.14,47.5 X4.28
L51
  Top 0.406: J9.51 329.67,216.16 330.88,217.38 338.38,217.38 339.62,216.12 342.27,216.12 J19.51
  Top 0.506: J19.51 343.04,216.16 344.25,217.38 365.5,217.38 398.25,184.62 435.75,184.62 467.75,216.62 479.81,216.62 J10.51 480.62,216.75 481.88,218 486.88,218 488.12,216.75 J20.51
  Top 0.51: J9.51 305.67,216.16 274.5,185 84.75,185 51.5,151.75 51.5,72.88 24.62,46 20.25,46 X4.10
L52
  Top 0.406: J9.52 338.33,216.16 339.62,214.88 343.12,214.88 344.38,216.12 344.81,216.12 J19.52 | J10.52 482.12,216.75 480.75,215.38 478.88,215.38
  Top 0.506: 81.75,180.38 52.75,151.38 52.75,72.38 25.12,44.75 23.13,44.75 X4.29 | 478.88,215.38 468,215.38 436.25,183.62 397.62,183.62 365,216.25 344.94,216.25 J19.52 | J10.52 486.88,216.75 488.12,215.5 493.43,215.5 J20.52
  Top 0.51: J9.52 331.04,216.16 329.75,214.88 305.75,214.88 274.88,184 85.38,184 81.75,180.38
L53
  Top 0.406: J9.53 329.62,213.62 330.88,214.88 338.62,214.88 339.88,213.62 J19.53
  Top 0.506: 82.12,178.75 54.12,150.75 54.12,72.12 25.38,43.38 25.25,43.38 25.12,43.25 20.23,43.25 X4.11 | J19.53 343.12,213.62 344.38,214.88 364.75,214.88 397.12,182.5 436.62,182.5 468.38,214.25 479.89,214.25 J10.53 480.7,214.21 482,215.5 486.75,215.5 488,214.25 492.09,214.25 J20.53
  Top 0.51: J9.53 306,213.62 275.38,183 86.38,183 82.12,178.75
L54
  Top 0.406: J9.54 338.88,213.62 340.12,212.38 342.88,212.38 344.12,213.62 J19.54
  Top 0.506: 86.38,181.25 55.5,150.38 55.5,71.75 25.62,41.88 23.08,41.88 X4.30 | J19.54 344.98,213.75 364.12,213.75 396.5,181.38 437,181.38 468.5,212.88 480.75,212.88 482.08,214.21 J10.54 486.8,214.21 488.12,212.88 493.35,212.88 J20.54
  Top 0.51: J9.54 331.12,213.62 329.88,212.38 306.25,212.38 275.88,182 87.12,182 86.38,181.25
L55
  Top 0.406: J9.55 329.83,211.09 331.12,212.38 339.12,212.38 340.38,211.12 342.27,211.12 J19.55
  Top 0.506: 87.5,180 56.75,149.25 56.75,71 26.25,40.5 20.24,40.5 X4.12 | J19.55 342.83,211.09 344.12,212.38 363.88,212.38 395.88,180.38 437.5,180.38 468.88,211.75 479.85,211.75 J10.55 480.67,211.66 481.88,212.88 486.75,212.88 488,211.62 492.1,211.62 J20.55
  Top 0.51: J9.55 306.83,211.09 276.25,180.5 88,180.5 87.5,180
L56
  Top 0.406: J9.56 339.42,211.09 340.75,209.75 342.88,209.75 344.12,211 344.76,211 J19.56
  Top 0.506: 88.88,177.88 58,147 58,70.62 26.5,39.12 X4.31 | 363.88,211 395.62,179.38 437.88,179.38 468.88,210.38 480.75,210.38 482.04,211.66 J10.56 486.46,211.66 487.75,210.38 492.62,210.38 493.88,211.62 494.63,211.62 J20.56 | 363.88,211 363.75,211.12 | J19.56 363.79,211.09 363.88,211
  Top 0.51: J9.56 331.08,211.09 329.75,209.75 307.75,209.75 277.12,179.12 90.12,179.12 88.88,177.88
L57
  Top 0.406: J9.57 329.92,208.54 331.12,209.75 339.62,209.75 340.75,208.62 342.23,208.62 J19.57
  Top 0.506: 90.12,176.62 59.25,145.75 59.25,70.25 26.75,37.75 X4.13 | J19.57 342.92,208.54 344.12,209.75 363.62,209.75 395,178.38 438.25,178.38 469.12,209.25 479.81,209.25 J10.57 480.62,209.12 481.88,210.38 486.62,210.38 487.88,209.12 J20.57
  Top 0.51: J9.57 308.3,208.54 277.5,177.75 91.25,177.75 90.12,176.62
L58
  Top 0.406: J9.58 339.7,208.54 341,207.25 342.88,207.25 344.12,208.5 344.81,208.5 J19.58
  Top 0.506: X4.32 27.24,36.36 60.75,69.88 60.75,145.38 91.38,176 | J19.58 344.93,208.62 363.12,208.62 394.38,177.38 438.62,177.38 469.12,207.88 480.75,207.88 482,209.12 J10.58 486.5,209.12 487.75,207.88 493.43,207.88 J20.58
  Top 0.51: J9.58 331.3,208.54 330,207.25 308.88,207.25 278.25,176.62 92,176.62 91.38,176
L59
  Top 0.406: J9.59 330,206 331.25,207.25 340,207.25 341.25,206 J19.59
  Top 0.506: 92.38,174.62 62.12,144.38 62.12,69.75 27.38,35 X4.14 | J19.59 342.88,206 344.12,207.25 362.88,207.25 393.75,176.38 439.25,176.38 469.38,206.5 479.85,206.5 J10.59 480.71,206.59 482,207.88 486.62,207.88 487.88,206.62 492.1,206.62 J20.59
  Top 0.51: J9.59 309.63,206 278.75,175.12 92.88,175.12 92.38,174.62
L60
  Top 0.406: J9.60 339.87,206 341.25,204.62 342.75,204.62 344.12,206 J19.60
  Top 0.506: 96.88,173.88 93.75,173.88 63.62,143.75 63.62,69.38 27.75,33.5 23.17,33.5 X4.33 | J19.60 362.5,206 393.12,175.38 439.75,175.38 469.75,205.38 480.62,205.38 481.83,206.59 J10.60 486.54,206.59 487.75,205.38 493,205.38 494.12,206.5 494.59,206.5 J20.60
  Top 0.51: J9.60 331.65,205.9 330.25,204.5 310.12,204.5 279.5,173.88 96.88,173.88
L61
  Top 0.506: X4.15 28.35,32.22 65.12,69 65.12,143.5 93.25,171.62 438,171.62 470.38,204 479.89,204 J10.61 480.67,204.04 481.88,205.25 486.62,205.25 487.88,204 492.09,204 J20.61
L62
  Top 0.506: X4.34 23.03,30.88 18.5,30.88 17.62,30 17.62,21.5 20,19.12 24.38,19.12 72.38,67.12 72.38,140.12 98.38,166.12 438.62,166.12 445.5,173 445.62,173 470.12,197.5 470.25,197.5 471.5,198.75 494.38,198.75 496.5,200.88 496.5,202.62 495.08,204.04 J20.62 493.38,202.75 487.62,202.75 486.33,204.04 J10.62
L63
  Top 0.506: X4.16 29.85,29.48 68.38,68 68.38,140.75 96.75,169.12 437.38,169.12 469.62,201.38 479.81,201.38 J10.63
  Bottom 0.506: J10.63 480.12,201.5 480.12,201.25 481.25,200.12 490.75,200.12 J20.63
L64
  Top 0.506: X4.35 23.09,28.12 31,28.12 70.12,67.25 70.12,140.62 97.25,167.75 438.38,167.75 470.62,200 480.75,200 482.25,201.5 J10.64 483.25,201.5 485,199.75 492.92,199.75 J20.64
